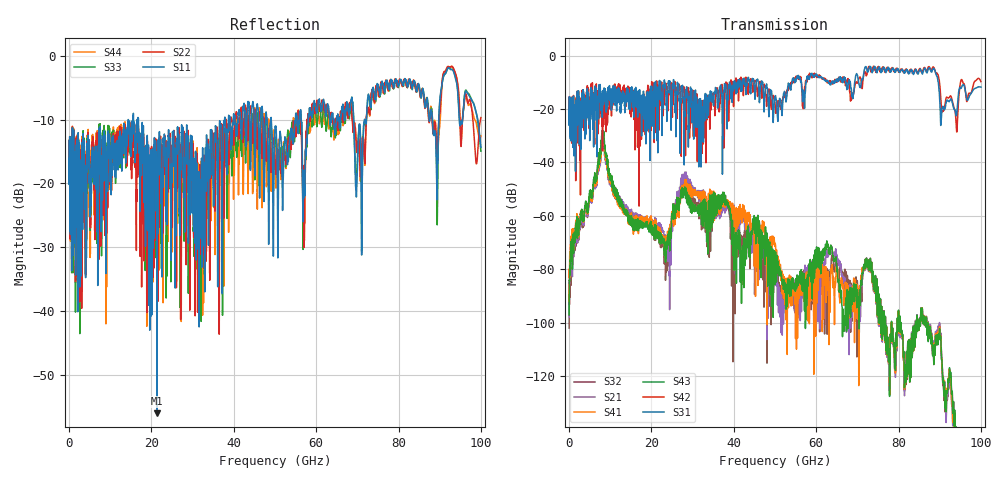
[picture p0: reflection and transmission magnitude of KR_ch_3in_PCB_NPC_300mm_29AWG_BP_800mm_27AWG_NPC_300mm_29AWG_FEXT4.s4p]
# GHz S RI R 45
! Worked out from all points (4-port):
!   4000 points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, 25 MHz to 100 GHz, reference 45 ohm
!   strongest paths, dB at 25 MHz, 25.02 GHz, 50.02 GHz, 75.03 GHz, 100 GHz:
!     S31: -20.6, -14.3, -15.8, -5.2, -11.8
!     S42: -20.6, -18.0, -18.0, -4.3, -9.8
!     S43: -97.2, -60.1, -82.8, -89.7, -173.7
!     S41: -92.1, -60.3, -70.6, -89.9, -174.3
!     S21: -98.0, -62.6, -79.0, -89.9, -175.9
!     S32: -102.0, -60.9, -81.6, -89.5, -173.8
!   lowest |S11| = -56.0 dB at 21.32 GHz (marker M1), VSWR 1.00, Z = 44.9 + j0.12 ohm
!   |S11| at or under -10 dB: start of sweep to 14.4 GHz; 16.85 GHz to 37.75 GHz (20.9 GHz wide, 76.6 % of centre); 49.1 GHz to 54.96 GHz (5.865 GHz wide, 11.3 % of centre)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
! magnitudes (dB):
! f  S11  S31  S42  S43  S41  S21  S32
! 25 MHz  -16.1  -20.6  -20.6  -97.2  -92.1  -98.0  -102.0
! 8.2 GHz  -18.7  -17.0  -26.6  -28.2  -30.1  -32.0  -29.7
! 21.32 GHz  -56.0  -20.7  -11.1  -66.7  -66.2  -63.9  -66.3
! 24.32 GHz  -14.6  -10.8  -14.6  -65.9  -65.8  -72.8  -69.0
! 27.95 GHz  -21.5  -40.9  -13.4  -51.7  -49.9  -47.0  -48.5
! 48.27 GHz  -13.9  -14.5  -13.4  -71.4  -72.8  -87.5  -75.0
! 100 GHz  -14.4  -11.8  -9.8  -173.7  -174.3  -175.9  -173.8
